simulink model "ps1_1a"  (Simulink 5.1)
settings: Solver=ode45  StartTime=0.0  StopTime=10.0  RelTol=1e-3
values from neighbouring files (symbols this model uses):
  d = 0.0001    [ps4_3.m]
  s = tf('s')    [ps7_3_2.m]    (also in ps4_2.m; ps7_1_2.m; ps4_3.m; ps2_3.m)
libraries: cstblocks x2

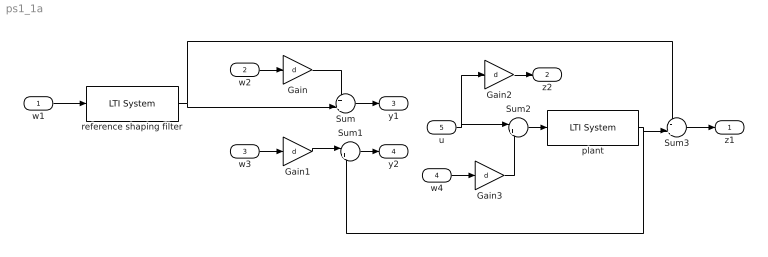
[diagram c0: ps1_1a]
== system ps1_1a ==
  w1 : Inport
  w2 : Inport  Port=2
  w3 : Inport  Port=3
  w4 : Inport  Port=4
  u : Inport  Port=5
  Gain{,1..3} (4 alike) : Gain  Gain=d
  Sum : Sum  Inputs=++|
  Sum1 : Sum  Inputs=|++
  Sum2 : Sum  Inputs=|++
  Sum3 : Sum  Inputs=-+|
  plant : cstblocks/LTI System  sys=s/(s^2+1)  IC=[]
  reference shaping filter : cstblocks/LTI System  sys=10/(s+10)  IC=[]
  z1 : Outport
  z2 : Outport  Port=2
  y1 : Outport  Port=3
  y2 : Outport  Port=4
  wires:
  w1/1 -> reference shaping filter/1
  w2/1 -> Gain/1
  Gain/1 -> Sum/1
  reference shaping filter/1 -> Sum/2, Sum3/1
  Gain1/1 -> Sum1/1
  w3/1 -> Gain1/1
  Gain2/1 -> z2/1
  Sum2/1 -> plant/1
  plant/1 -> Sum3/2, Sum1/2
  Sum3/1 -> z1/1
  Sum/1 -> y1/1
  Sum1/1 -> y2/1
  w4/1 -> Gain3/1
  u/1 -> Sum2/1, Gain2/1
  Gain3/1 -> Sum2/2
